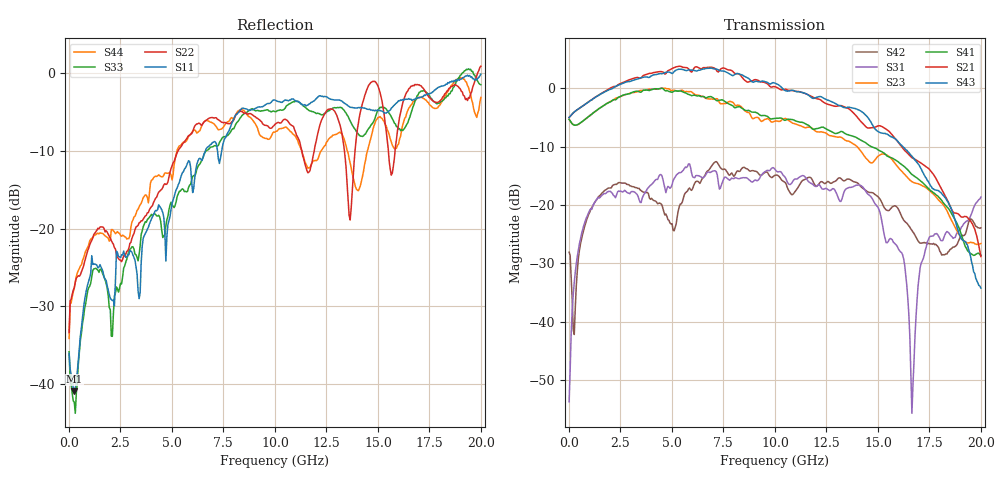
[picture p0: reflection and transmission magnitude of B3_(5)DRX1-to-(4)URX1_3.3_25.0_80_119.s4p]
!Agilent Technologies,N5225A,MY51451112,A.09.50.13
!Agilent N5225A: A.09.50.13
!Date: Sunday, March 12, 2017 05:21:57
!Correction: S11(Full 4 Port(1,2,3,4))
!S12(Full 4 Port(1,2,3,4))
!S13(Full 4 Port(1,2,3,4))
!S14(Full 4 Port(1,2,3,4))
!S21(Full 4 Port(1,2,3,4))
!S22(Full 4 Port(1,2,3,4))
!S23(Full 4 Port(1,2,3,4))
!S24(Full 4 Port(1,2,3,4))
!S31(Full 4 Port(1,2,3,4))
!S32(Full 4 Port(1,2,3,4))
!S33(Full 4 Port(1,2,3,4))
!S34(Full 4 Port(1,2,3,4))
!S41(Full 4 Port(1,2,3,4))
!S42(Full 4 Port(1,2,3,4))
!S43(Full 4 Port(1,2,3,4))
!S44(Full 4 Port(1,2,3,4))
!S4P File: Measurements: <S11,S12,S13,S14>,
!<S21,S22,S23,S24>,
!<S31,S32,S33,S34>,
!<S41,S42,S43,S44>:
# Hz S  dB  R 50
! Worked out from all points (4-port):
!   401 points, 10 MHz to 20 GHz, reference 50 ohm
!   strongest paths, dB at 10 MHz, 5.008 GHz, 10.01 GHz, 15 GHz, 20 GHz:
!     S43: -5.0, 2.5, 0.9, -7.4, -34.2
!     S21: -5.0, 3.3, 0.2, -6.5, -28.8
!     S41: -5.3, -0.7, -5.2, -10.5, -28.6
!     S23: -5.3, -0.4, -5.6, -11.7, -26.6
!     S31: -53.7, -16.5, -13.9, -20.4, -18.6
!     S42: -28.1, -23.2, -14.9, -18.6, -23.9
!   lowest |S11| = -40.9 dB at 259.9 MHz (marker M1), VSWR 1.02, Z = 50.3 - j0.865 ohm
!   |S11| at or under -10 dB: start of sweep to 6.632 GHz; 7.211 GHz to 7.419 GHz (207.5 MHz wide, 2.84 % of centre)
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1e7  -36.03 -38.7  -67.51 161.0  -51.72 17.0  -63.56 139.5
     -5.02 1.6  -33.36 39.2  -5.33 -179.8  -27.94 38.0
     -53.67 17.0  -64.67 115.3  -35.82 -45.9  -66.34 115.6
     -5.33 -179.8  -28.07 38.1  -5.00 1.7  -34.11 45.2
2.59875e8  -40.88 -72.4  -49.84 54.7  -33.15 94.6  -50.60 52.8
           -4.08 0.1  -27.60 -131.8  -6.33 172.6  -41.64 -161.8
           -33.22 95.5  -50.11 57.2  -42.28 -78.8  -50.38 55.3
           -6.32 171.9  -42.15 -169.5  -4.07 -0.7  -27.65 -137.9
5.157425e9  -15.43 88.3  -37.81 12.2  -15.49 28.8  -39.49 -18.3
            3.60 171.0  -11.00 143.9  -0.40 -26.9  -24.25 57.6
            -15.24 26.9  -37.64 1.6  -17.03 103.8  -38.68 -54.9
            -0.48 -42.6  -23.81 59.3  2.98 161.1  -11.02 122.9
8.255875e9  -5.02 36.7  -39.73 -109.5  -15.69 0.2  -36.41 -138.6
            2.42 17.7  -5.04 80.8  -2.94 -166.0  -13.86 47.1
            -15.50 -0.6  -32.45 -115.9  -6.07 58.4  -31.74 -151.9
            -3.15 170.9  -14.25 50.3  2.45 5.0  -4.85 45.6
1.215392e10  -2.98 -17.6  -33.37 -149.2  -16.11 -21.2  -34.62 170.4
             -1.90 -149.2  -7.01 66.8  -7.50 29.9  -16.05 40.3
             -16.50 -20.2  -34.10 -142.0  -5.25 -3.5  -33.16 175.1
             -6.83 -5.8  -16.30 43.2  -1.43 -173.4  -10.56 -6.3
1.665168e10  -3.55 -76.2  -34.74 122.8  -47.91 4.0  -36.69 86.7
             -11.89 9.7  -1.71 63.5  -16.01 166.7  -24.49 54.4
             -55.64 21.5  -33.05 122.1  -4.85 -81.3  -32.98 87.5
             -14.77 114.3  -24.33 54.5  -11.64 -38.8  -4.06 -61.8
2e10  -0.18 -114.1  -33.00 62.8  -18.67 121.3  -35.61 21.6
      -28.82 -149.6  0.84 17.1  -26.58 30.9  -23.90 102.0
      -18.64 121.3  -33.97 40.5  -1.54 -87.7  -35.25 -7.7
      -28.60 -14.7  -23.90 102.7  -34.21 -177.0  -3.18 -136.6
